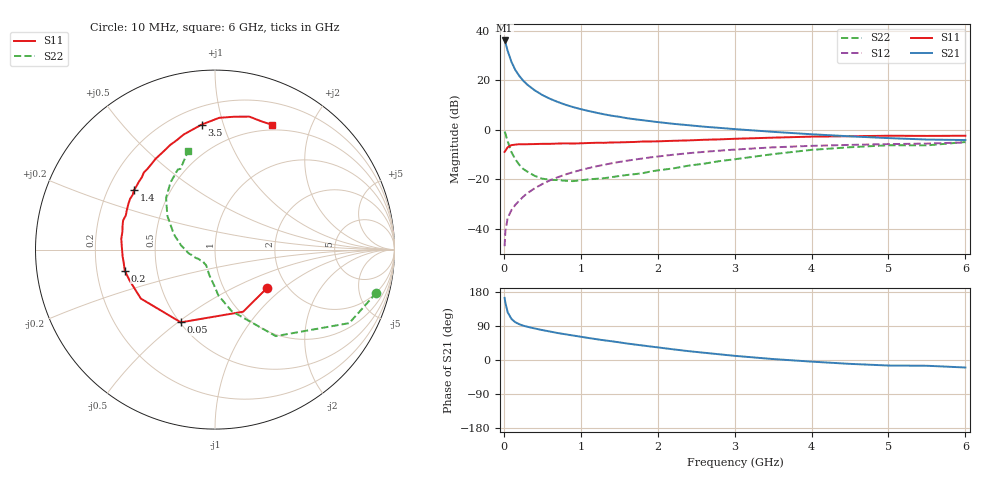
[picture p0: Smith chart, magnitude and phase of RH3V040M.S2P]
! SIEMENS Small Signal Semiconductors
! BFR106
! Si NPN RF Bipolar Junction Transistor in SOT23
! VCE = 3 V  IC = 40 mA
! Common Emitter S-Parameters:  August  1996
# GHz  S  MA  R  50
!  f  S11  S21  S12  S22
! GHz  MAG  ANG  MAG  ANG  MAG  ANG  MAG  ANG
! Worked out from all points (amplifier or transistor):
!   36 points, 10 MHz to 6 GHz, reference 50 ohm
!   highest |S21| = 36.2 dB at 10 MHz (marker M1)
!   |S21| within 3 dB of that: start of sweep to 39.1 MHz
!   unconditionally stable (mu >= 1): 259 MHz to 2.429 GHz; 5.453 GHz to 5.713 GHz
!   at 250 MHz: K = 1.00, MSG = 23.5 dB, |S12| = -27.0 dB
!   at 1.4 GHz: K = 1.06, MAG = 8.1 dB, |S12| = -13.5 dB
!   at 6 GHz: K = 1.00, MSG = 0.5 dB, |S12| = -5.0 dB
!   S11 on the Smith chart (normalised r, x): 10 MHz: 1.59, -0.78; 50 MHz: 0.51, -0.51; 200 MHz: 0.32, -0.10; 1.4 GHz: 0.31, +0.30; 3.5 GHz: 0.31, +0.85; 6 GHz: 0.44, +1.46
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0.01  0.3606 -36.2  64.37 163.9  0.0045 80.0  0.9305 -15.0
0.02  0.38 -65.6  58.34 151.1  0.009 70.6  0.8528 -28.7
0.05  0.448 -115.2  39.58 125.8  0.0167 59.8  0.5892 -54.9
0.1  0.4952 -146.6  23.5 108.1  0.0243 58.9  0.3547 -74.9
0.15  0.5059 -160.0  16.26 99.5  0.0308 61.5  0.2546 -85.9
0.2  0.5163 -166.9  12.44 94.5  0.0374 65.0  0.1992 -91.4
0.25  0.5138 -172.4  9.988 90.7  0.0446 67.0  0.1639 -97.9
0.3  0.5162 -175.8  8.369 88.0  0.0521 68.5  0.1459 -102.4
0.4  0.5198 177.8  6.348 83.3  0.0664 70.1  0.1187 -110.6
0.5  0.5257 173.5  5.088 79.0  0.081 70.3  0.104 -116.8
0.6  0.5253 169.2  4.27 75.1  0.0962 69.9  0.0987 -121.7
0.7  0.5318 165.5  3.694 71.2  0.111 69.2  0.0972 -127.2
0.8  0.5372 162.4  3.242 67.9  0.1261 68.1  0.0945 -132.7
1.1  0.5458 152.1  2.42 58.1  0.1699 64.6  0.1007 -143.7
1.4  0.5598 143.8  1.946 49.5  0.2121 60.3  0.1116 -154.0
1.7  0.5729 135.4  1.649 40.9  0.2526 55.9  0.1282 -165.0
2.2  0.6047 123.1  1.335 28.2  0.3163 48.0  0.1673 179.7
2.8  0.6462 109.1  1.105 15.1  0.3821 38.5  0.2347 161.5
3.5  0.7005 96.1  0.918 2.5  0.4462 27.8  0.3256 144.6
4.5  0.7485 81.6  0.745 -10.2  0.5002 13.1  0.4483 123.6
5.5  0.7599 69.8  0.641 -15.2  0.5317 3.9  0.4891 113.2
6  0.7648 65.5  0.627 -19.8  0.5614 -3.2  0.5706 105.2
